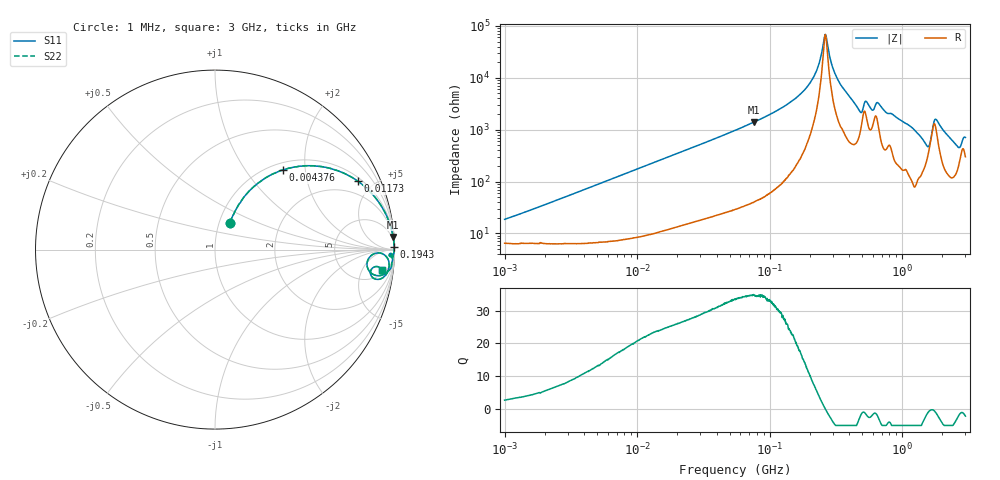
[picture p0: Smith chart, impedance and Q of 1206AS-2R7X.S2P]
!s-Parameter Generated by FASTRON Sdn. Bhd.
!FASTRON P/N : 1206AS-2R7X
!Keysight Technologies: E4991B_MY54100416_A.01.15
!Date created: Thu Nov 16 13:51:45 2023
!Version  : Rev00 Thu Nov 16 13:51:45 2023
!Data & Calibration Information:
!Freq	S11	S21	S12	S22
!PortZ  Port1:50+j0  Port2:50+j0
!When reading reference impedance value at option line is always used.
! Remarks : This data is being provided solely for informational purposes.
# Hz S dB R 50
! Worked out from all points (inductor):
!   1601 points, 1 MHz to 3 GHz, reference 50 ohm
!   read as one part in series: L = 2.78 uH near 1.094 MHz
!   highest Q = 34.7 at 76.59 MHz (marker M1), where L = 2.92 uH
!   self-resonance near 262.3 MHz
!   S11 on the Smith chart (normalised r, x): 1 MHz: 1.13, +0.35; 4.376 MHz: 1.13, +1.53; 11.73 MHz: 1.18, +4.07; 194.3 MHz: open; 3 GHz: 7, -13
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1000000  -15.24 60.4  -0.66 -9.3  -0.66 -9.3  -15.24 60.4
3804036  -5.49 52.6  -1.96 -32.0  -1.96 -32.0  -5.49 52.6
4376170  -4.66 49.5  -2.35 -35.6  -2.35 -35.6  -4.66 49.5
1.172775e7  -1.09 25.6  -7.27 -61.8  -7.27 -61.8  -1.09 25.6
1.447069e7  -0.76 21.4  -8.75 -66.2  -8.75 -66.2  -0.76 21.4
5.477226e7  -0.07 5.9  -19.77 -82.4  -19.77 -82.4  -0.07 5.9
7.658877e7  -0.04 4.1  -22.98 -84.3  -22.98 -84.3  -0.04 4.1
1.375402e8  -0.02 1.8  -29.95 -85.9  -29.95 -85.9  -0.02 1.8
1.942587e8  -0.01 0.8  -36.87 -84.2  -36.87 -84.2  -0.01 0.8
2.083556e8  -0.01 0.6  -39.13 -82.9  -39.13 -82.9  -0.01 0.6
2.314421e8  -0.01 0.3  -44.17 -77.5  -44.17 -77.5  -0.01 0.3
2.636002e8  -0.01 -0.0  -56.69 1.3  -56.69 1.3  -0.01 -0.0
3.220132e8  -0.02 -0.6  -39.96 79.1  -39.96 79.1  -0.02 -0.6
4.733803e8  -0.12 -2.3  -27.57 69.6  -27.57 69.6  -0.12 -2.3
5.337858e8  -0.13 -1.4  -31.06 56.9  -31.06 56.9  -0.13 -1.4
5.929311e8  -0.17 -2.1  -27.75 60.6  -27.75 60.6  -0.17 -2.1
6.553423e8  -0.11 -1.6  -30.47 64.8  -30.47 64.8  -0.11 -1.6
7.925923e8  -0.11 -2.7  -26.31 73.3  -26.31 73.3  -0.11 -2.7
1.534307e9  -0.99 -8.9  -14.78 49.4  -14.78 49.4  -0.99 -8.9
1.791767e9  -0.38 -2.5  -24.40 44.1  -24.40 44.1  -0.38 -2.5
2.594767e9  -0.71 -10.4  -14.40 60.6  -14.40 60.6  -0.71 -10.4
3e9  -0.57 -6.9  -17.58 58.1  -17.58 58.1  -0.57 -6.9
